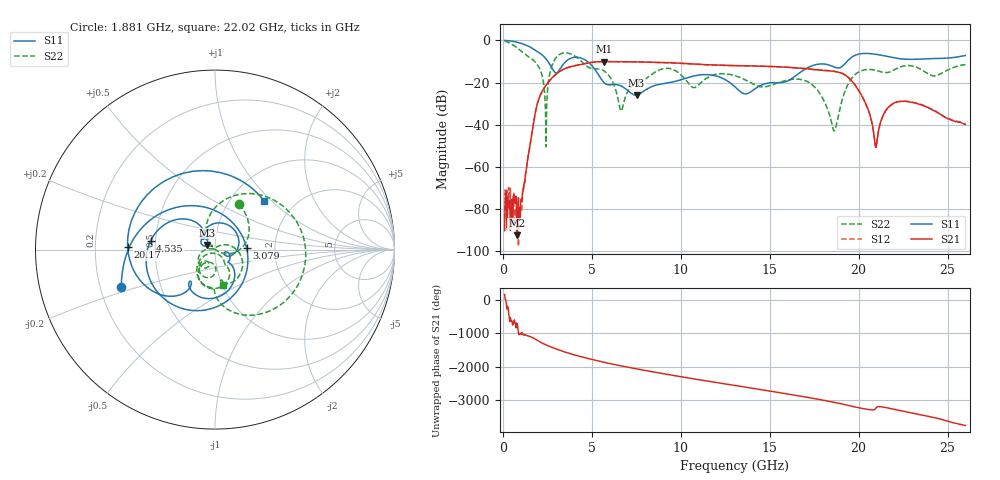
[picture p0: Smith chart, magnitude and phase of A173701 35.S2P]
!  2-Port S-parameters saved by WinCal
! VAR MeasName=S-Parameters (CALIBRATED_DATA) read from VNA (N5245A)
! VAR MeasDate=2017-6-7 10:30:46
! VAR NAME=A173701 35
! VAR FILENAME=A173701 35.S2P
! VAR DATE=2017-6-7 10:30:46
! VAR PHYS_PORTS=1,2
# Hz S DB R 50
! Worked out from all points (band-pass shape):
!   801 points, 100 MHz to 26 GHz, reference 50 ohm
!   highest |S21| = -10.00 dB at 5.668 GHz (marker M1); lowest = -92.4 dB at 779.9 MHz (marker M2)
!   |S21| within 3 dB of the highest: 3.604 GHz to 16.4 GHz (12.8 GHz wide, 128 % of centre)
!   lowest |S11| = -25.9 dB at 7.514 GHz (marker M3), VSWR 1.11, Z = 45.8 + j2.41 ohm
!   |S11| at or under -10 dB: 2.536 GHz to 3.539 GHz (1.003 GHz wide, 33 % of centre); 4.757 GHz to 19.34 GHz (14.59 GHz wide, 121 % of centre)
!   |S22| runs from -50.4 to -0.2 dB; largest |S21 - S12| = 0.0048
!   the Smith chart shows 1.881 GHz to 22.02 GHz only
!   S11 on the Smith chart (normalised r, x): 1.881 GHz: 0.29, -0.18; 3.079 GHz: 1.43, +0.03; 4.535 GHz: 0.47, +0.05; 20.17 GHz: 0.35, +0.01; 22.02 GHz: 1.42, +0.90
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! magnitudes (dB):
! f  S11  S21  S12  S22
! 100 MHz  0.0  -90.2  -84.8  -0.2
! 779.9 MHz  -0.8  -92.4  -81.0  -3.4
! 1.039 GHz  -1.4  -75.1  -79.9  -5.1
! 1.881 GHz  -5.0  -32.1  -32.0  -10.9
! 2.431 GHz  -8.8  -21.2  -21.2  -50.4
! 3.079 GHz  -15.1  -15.4  -15.4  -7.4
! 4.438 GHz  -8.5  -11.3  -11.3  -10.1
! 4.535 GHz  -8.8  -11.1  -11.1  -10.8
! 5.668 GHz  -19.8  -10.0  -10.0  -14.4
! 6.64 GHz  -21.5  -10.1  -10.1  -33.4
! 7.514 GHz  -25.9  -10.2  -10.2  -20.5
! 8.744 GHz  -20.9  -10.5  -10.5  -14.2
! 10.72 GHz  -16.9  -11.2  -11.2  -22.4
! 13.05 GHz  -22.0  -11.9  -11.9  -16.8
! 17.39 GHz  -12.0  -13.8  -13.6  -21.0
! 18.65 GHz  -12.7  -14.7  -14.7  -42.7
! 19.36 GHz  -9.8  -17.2  -17.0  -21.5
! 20.17 GHz  -6.3  -26.1  -26.2  -14.3
! 20.95 GHz  -6.6  -50.3  -50.7  -14.2
! 21.69 GHz  -7.8  -31.5  -31.6  -15.1
! 22.02 GHz  -8.3  -29.5  -29.7  -13.9
! 26 GHz  -7.2  -39.8  -39.7  -11.5
